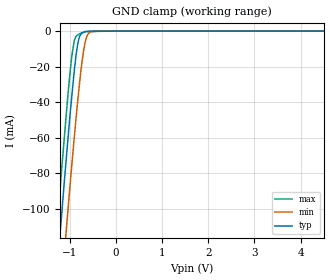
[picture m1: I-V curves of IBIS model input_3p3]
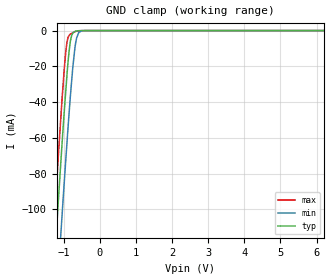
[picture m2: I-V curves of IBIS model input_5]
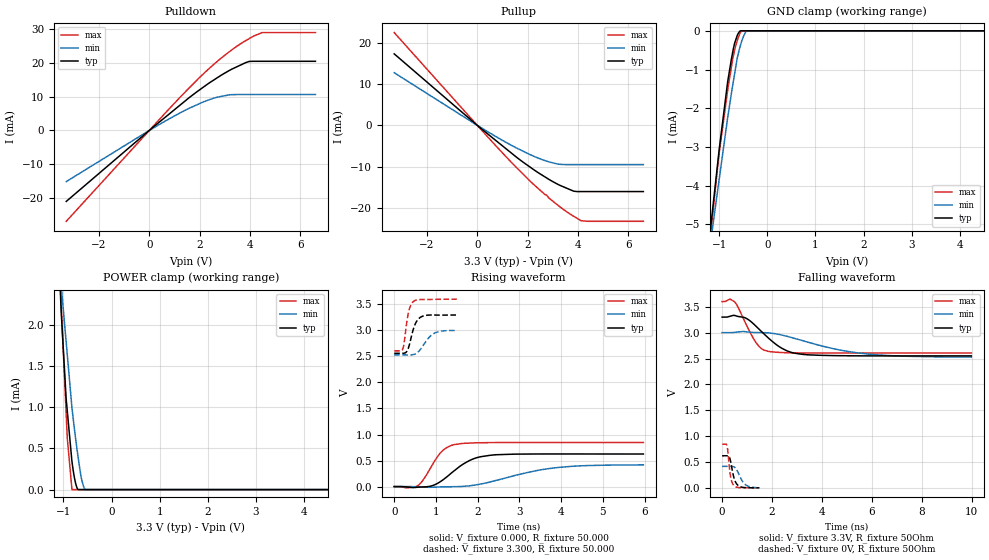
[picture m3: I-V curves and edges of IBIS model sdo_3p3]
|Texas Instruments Incorporated
| 2.7V-5.5V, 10 bit, 3MSPS, Serial ADC
| Marketing part#   Digital Voltage Range   Package-type   #pins
| ADS7884SDBVR   2.7V to 5.5V   SOT-23   6
| ADS7884SDBVT   2.7V to 5.5V   SOT-23   6
[IBIS Ver]   3.2
[File name]   ads7884.ibs
|SIMDE Ver   V3.0 - 201101 - RHL4 - Build 450
[File Rev]   1.0
[Date]   3/20/2011
[Source]
| Texas Instruments Incorporated.
| Analog-eLab Design Center, HPA
| 12500 TI Blvd
| Dallas, TX -75243
| e-mail: elab_ibis@list.ti.com
[Notes]   Revision History:
| Rev 1.0: 3/20/2011
| - Initial version of the model
| - Model generated from simulations in TISPICE
| - Model matched to SPICE simulation
| - C_comp although listed in numerical order of value are
|   obtained from varying PVT conditions. For PVT conditions for
|   each specific value refer the buffer description under
|   respective [Model]. IBIS model user is responsible for using
|   appropriate C_comp to simulate for Signal Integrity.
| - Model names with a trailing _3p3 contains the model for
|   3.3V [3.0V and 3.6V].Model names with a trailing _5 contains
|   the model for 5.0V [4.5V and 5.5V].
| - Rleative of ADS7883
[Disclaimer]
| This model is designed as an aid for customers of Texas Instruments.
| TI and its licensors and suppliers make no warranties, either expressed
| or implied, with respect to this  model, including the warranties of
| merchantability or fitness for a particular purpose. The model is
| provided solely on an "as is" basis. The entire risk as to its quality
| and performance is with the customer.
[Copyright]
 (C) Copyright 2011 Texas Instruments Incorporated.All rights reserved.
|   ADS7884
[Component]   ADS7884
[Manufacturer]   TI
[Package]   |6 SOT-23  -  DBV package
|   typ   min   max
R_pkg   0.00833   0.00820   0.00840
L_pkg   0.95512nH   0.93518nH   0.96766nH
C_pkg   0.21252pF   0.20183pF   0.24256pF
[Pin]  signal_name   model_name   R_pin   L_pin   C_pin
1   VDD   POWER   0.00811   0.93717nH  0.21052pF
2   GND   GND   0.00820   0.89025nH  0.21719pF
3   VIN   TERM   0.00840   0.96766nH  0.20183pF
4   SCLK   INPUT   0.00831   0.95468nH  0.20385pF
5   SDO   SDO   0.00820   0.93518nH  0.24256pF
6   _CS   INPUT   0.00840   0.96296nH  0.20183pF
|   Model Selectors
[Model Selector] INPUT
input_3p3   3.3V digital input
input_5   5.0V digital input
[Model Selector] SDO
sdo_3p3   3.3V digital 3-state output
sdo_5   5.0V digital 3-state output
[Model Selector] TERM
term_3-3V   3.3V nominal termination
term_5-0V   5.0V nominal termination
[Model]  term_3-3V
Model_type Terminator
C_comp   1.0e-20F  1.0e-20F  1.0e-20F
|   typ   min   max
[Voltage Range]   3.3V   3.0V   3.6V
[POWER Clamp Reference]   3.3V   3.0V   3.6V
[GND Clamp Reference]   0V   0V   0V
|Ambient Temperature   25   125   -40
|Junction Temperature
[Temperature Range]   30   130   -40
[Model]  term_5-0V
Model_type Terminator
C_comp   1.0e-20F  1.0e-20F  1.0e-20F
|   typ   min   max
[Voltage Range]   5.0V   4.5V   5.5V
[POWER Clamp Reference]   5.0V   4.5V   5.5V
[GND Clamp Reference]   0V   0V   0V
|Ambient Temperature   25   125   -40
|Junction Temperature
[Temperature Range]   30   130   -40
| Models and submodels in the file (6): input_3p3 (Input), input_5 (Input), sdo_3p3 (3-state), sdo_5 (3-state), term_3-3V (Terminator), term_5-0V (Terminator)
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|   input_3p3 Model
[Model]   input_3p3
Model_type   Input
Vinl = 0.4
Vinh = 1.5
|   typ   min   max
|   (nom PVT)   (Fast PVT)   (slow PVT)
|C_comp from frequency sweep method (F=48MHz)
|Average
C_comp   9.883e-13   8.635e-13   1.118e-12
|C_comp from LC tank measurement(L=1nH)
|Resonant Frequency(Hz)   5.810e+09   6.010e+09   5.610e+09
|C_comp   7.511e-13   7.020e-13   8.056e-13
| Where nom  PVT is Nominal Process,  3.3V,  30C
|   Fast PVT is Strong Process,   3.6V,  -40C
|   Slow PVT is Weak Process,   3V,  130C
[Voltage Range]   3.3   3   3.6
|Ambient Temperature   25   125   -40
|Junction Temperature
[Temperature Range]   30   130   -40
[Power Clamp Reference]   3.3   3   3.6
[GND Clamp Reference]   0   0   0
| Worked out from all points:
|   GND clamp passes 1 mA (typ) near -0.73 V on its own axis
[GND Clamp]
|   Voltage   I(typ)   I(min)   I(max)
-3.3V     -824.7mA   -854.6mA   -807mA
-1.294V   -141.5mA   -182mA     -117mA
-1.167V   -100.8mA   -140.8mA   -75.49mA
-1.115V   -84.28mA   -124.8mA   -59.63mA
-1.037V   -60.45mA   -100.3mA   -35.47mA
-954mV    -36.58mA   -75.2mA    -13.96mA
-896.4mV  -21.14mA   -58.46mA   -4.929mA
-802.8mV  -4.674mA   -33.3mA    -1.741mA
-741mV    -1.172mA   -18.82mA   -1.098mA
-666mV    -306.2uA   -6.367mA   -434.3uA
-540mV    -191.2uA   -375.4uA   -33.33uA
6.6V      0A         0A         0A
[POWER Clamp]
|   Voltage   I(typ)   I(min)   I(max)
-3.3V     0A         0A         0A
6.6V      0A         0A         0A
|   input_5 Model
[Model]   input_5
Model_type   Input
Vinl = 0.8
Vinh = 2.2
|   typ   min   max
|   (nom PVT)   (Fast PVT)   (slow PVT)
|C_comp from frequency sweep method (F=48MHz)
|Average
C_comp   9.397e-13   8.279e-13   1.058e-12
|C_comp from LC tank measurement(L=1nH)
|Resonant Frequency(Hz)   5.880e+09   6.070e+09   5.700e+09
|C_comp   7.334e-13   6.882e-13   7.804e-13
| Where nom  PVT is Nominal Process,  5V,  30C
|   Fast PVT is Strong Process,   5.5V,  -40C
|   Slow PVT is Weak Process,   4.5V,  130C
[Voltage Range]   5   4.5   5.5
|Ambient Temperature   25   125   -40
|Junction Temperature
[Temperature Range]   30   130   -40
[Power Clamp Reference]   5   4.5   5.5
[GND Clamp Reference]   0   0   0
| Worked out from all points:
|   GND clamp passes 1 mA (typ) near -0.74 V on its own axis
[GND Clamp]
|   Voltage   I(typ)   I(min)   I(max)
-5V       -1.412A    -1.436A    -1.399A
-1.368V   -166mA     -205.4mA   -141.5mA
-1.188V   -107.6mA   -147.5mA   -82.23mA
-1.127V   -88.16mA   -128.6mA   -62.97mA
-1.05V    -64.35mA   -104.5mA   -39.47mA
-979mV    -43.28mA   -82.7mA    -19.79mA
-913mV    -25.38mA   -63.22mA   -6.748mA
-815mV    -5.773mA   -36.27mA   -1.956mA
-670mV    -322.9uA   -6.853mA   -476uA
-580.5mV  -63.28uA   -988.6uA   -181.1uA
-373.5mV  -1.333uA   -5.052uA   -6.916uA
10V       0A         0A         0A
[POWER Clamp]
|   Voltage   I(typ)   I(min)   I(max)
-5V       0A         0A         0A
10V       0A         0A         0A
|   sdo_3p3 Model
[Model]   sdo_3p3
Model_type   3-state
Polarity   Non-Inverting
Vmeas = 1.65
Vref = 1.65
Cref = 10pF
Rref = 50
|   typ   min   max
|   (nom PVT)   (Fast PVT)   (slow PVT)
|C_comp from frequency sweep method(F=48MHz)
|C_comp   9.342e-13   8.281e-13   1.130e-12
|ON state : BUFFER OUTPUT TURNED HIGH
|C_comp   9.342e-13   8.281e-13   1.130e-12
|OFF state: BUFFER IN HIGH IMPEDANCE
|C_comp   1.178e-12   9.982e-13   1.365e-12
|C_comp from LC tank measurement(L=1nH)
|Resonant Frequency(Hz)   6.460e+09   6.710e+09   6.330e+09
C_comp   6.076e-13   5.632e-13   6.328e-13
|ON state : BUFFER OUTPUT TURNED HIGH
|Resonant Frequency(Hz)   6.460e+09   6.710e+09   6.330e+09
|C_comp   6.076e-13   5.632e-13   6.328e-13
|OFF state: BUFFER IN HIGH IMPEDANCE
|Resonant Frequency   6.110e+09   6.600e+09   5.830e+09
|C_comp   6.792e-13   5.821e-13   7.460e-13
| Where nom  PVT is Nominal Process,  3.3V,  30C
|   Fast PVT is Strong Process,   3.6V,  -40C
|   Slow PVT is Weak Process,   3V,  130C
[Voltage Range]   3.3   3   3.6
|Ambient Temperature   25   125   -40
|Junction Temperature
[Temperature Range]   30   130   -40
[Pullup Reference]   3.3   3   3.6
[Pulldown Reference]   0   0   0
[Power Clamp Reference]   3.3   3   3.6
[GND Clamp Reference]   0   0   0
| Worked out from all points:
|   slope of the pulldown table from 0 to 0.495 V, typ, clamps not added: 162 ohm
|   slope of the pullup table from 0 to 0.495 V, typ, clamps not added: 200 ohm
|   GND clamp passes 1 mA (typ) near -0.78 V on its own axis
|   POWER clamp passes 1 mA (typ) near -0.93 V on its own axis
|   falling waveform, V_fixture 3.3V, R_fixture 50Ohm: 20-80 % time 1.08ns typ, 2.46ns min, 635ps max; typ from 3.3 V to 2.55 V
|   rising waveform, V_fixture 0.000, R_fixture 50.000: 20-80 % time 644ps typ, 1.33ns min, 413ps max; typ from 0 V to 0.625 V
|   rising waveform, V_fixture 3.300, R_fixture 50.000: 20-80 % time 162ps typ, 272ps min, 114ps max; typ from 2.56 V to 3.29 V
|   falling waveform, V_fixture 0V, R_fixture 50Ohm: 20-80 % time 180ps typ, 287ps min, 123ps max; typ from 0.621 V to 0.002 V
[Pulldown]
|   Voltage   I(typ)   I(min)   I(max)
-3.3V     -21.06mA   -15.19mA   -26.96mA
0V        0A         0A         0A
1.29V     7.925mA    5.45mA     10.38mA
2.277V    13.53mA    8.822mA    17.68mA
2.7V      15.62mA    9.857mA    20.48mA
3.27V     18.14mA    10.6mA     23.86mA
3.97V     20.45mA    10.65mA    27.23mA
4.483V    20.49mA    10.65mA    29.02mA
6.6V      20.49mA    10.65mA    29.02mA
[GND Clamp]
|   Voltage   I(typ)   I(min)   I(max)
-3.3V     -31.86mA   -26.3mA    -39mA
-1.18V    -5.077mA   -5.443mA   -5.263mA
-1.01V    -3.162mA   -3.913mA   -3.234mA
-825mV    -1.313mA   -2.237mA   -1.529mA
-726mV    -584.3uA   -1.442mA   -763.6uA
-683.1mV  -331.7uA   -1.122mA   -511uA
-630mV    -133.7uA   -725.1uA   -269.5uA
-567.6mV  -2.719uA   -407.5uA   -62.56uA
-535.2mV  0A         -273.4uA   0A
-486mV    0A         -111.5uA   0A
-438mV    0A         -1.634uA   0A
6.6V      0A         0A         0A
[Pullup]
|   Voltage   I(typ)   I(min)   I(max)
-3.3V     17.35mA    12.77mA    22.52mA
0V        0A         0A         0A
1.149V    -5.708mA   -4.153mA   -7.649mA
1.574V    -7.808mA   -5.548mA   -10.34mA
2.277V    -10.9mA    -7.585mA   -14.55mA
2.7V      -12.56mA   -8.577mA   -16.85mA
2.755V    -12.76mA   -8.682mA   -16.91mA
2.842V    -13.1mA    -8.851mA   -17.62mA
3.205V    -14.33mA   -9.386mA   -19.41mA
3.831V    -15.98mA   -9.532mA   -22.07mA
4.134V    -16.08mA   -9.532mA   -23.17mA
6.6V      -16.08mA   -9.532mA   -23.29mA
[POWER Clamp]
|   Voltage   I(typ)   I(min)   I(max)
-3.3V     43.14mA    33.87mA    53.61mA
-1.143V   3.495mA    3.12mA     4.243mA
-1.049V   2.194mA    2.498mA    2.361mA
-1.036V   2.045mA    2.406mA    2.099mA
-943.8mV  1.104mA    1.795mA    926.4uA
-920.4mV  955.6uA    1.64mA     627.4uA
-823.2mV  344uA      996.3uA    0A
-759mV    107.9uA    676.4uA    0A
-706.2mV  6.277uA    441.7uA    0A
-630mV    0A         145.2uA    0A
-555mV    0A         31.3nA     0A
6.6V      0A         0A         0A
[Ramp]
R_load = 50
|   typ   min   max
dV/dt_r   0.37497/6.43447e-10   0.250507/1.33256e-09   0.5127/4.11078e-10
dV/dt_f   0.449324/1.08338e-09   0.283649/2.45466e-09   0.595524/6.34571e-10
[Falling Waveform]
V_fixture = 3.3V
V_fixture_min = 3V
V_fixture_max = 3.6V
R_fixture = 50Ohm
|   Time   V(typ)   V(min)   V(max)
0s        3.3V       3V         3.6V
310ps     3.315V     3V         3.647V
510ps     3.331V     3.005V     3.588V
960ps     3.278V     3.017V     3.162V
1.34ns    3.132V     3.002V     2.822V
1.86ns    2.894V     2.995V     2.637V
2.6ns     2.648V     2.929V     2.612V
3.29ns    2.577V     2.836V     2.606V
5.88ns    2.551V     2.584V     2.606V
9.99ns    2.551V     2.527V     2.607V
[Rising Waveform]
V_fixture = 0.000
V_fixture_min = 0.000
V_fixture_max = 0.000
R_fixture = 50.000
|  time   V(typ)   V(min)   V(max)
0s        -2.813uV   8.632uV    0V
310ps     -7.985mV   158.5uV    -24.09mV
570ps     -11.73mV   -4.704mV   21.65mV
720ps     -6.205mV   -10.13mV   158mV
1.09ns    85.97mV    -6.545mV   631.3mV
1.45ns    311.3mV    -1.882mV   808.3mV
1.87ns    524mV      21.68mV    838.1mV
2.41ns    610mV      111.9mV    845.3mV
3.9ns     626.5mV    364.6mV    846mV
5.97ns    625.4mV    417.1mV    845.4mV
[Rising Waveform]
V_fixture = 3.300
V_fixture_min = 3.000
V_fixture_max = 3.600
R_fixture = 50.000
|  time   V(typ)   V(min)   V(max)
0s        2.559V     2.529V     2.606V
205ps     2.56V      2.529V     2.644V
235ps     2.562V     2.529V     2.746V
307ps     2.599V     2.528V     3.187V
346ps     2.675V     2.528V     3.357V
403ps     2.854V     2.529V     3.493V
478ps     3.069V     2.54V      3.565V
643ps     3.259V     2.65V      3.594V
955ps     3.295V     2.942V     3.595V
1.498ns   3.295V     2.998V     3.6V
[Falling Waveform]
V_fixture = 0V
V_fixture_min = 0V
V_fixture_max = 0V
R_fixture = 50Ohm
|   Time   V(typ)   V(min)   V(max)
0s        621.2mV    416.6mV    845.4mV
193ps     621.8mV    416.4mV    820.7mV
229ps     621mV      416.4mV    712mV
277ps     605.9mV    416.6mV    463.9mV
337ps     521.5mV    417.1mV    225.9mV
394ps     377mV      416.2mV    112.3mV
469ps     205.9mV    407.5mV    47.51mV
637ps     49.52mV    300.6mV    9.065mV
937ps     5.18mV     63.17mV    2.442mV
1.498ns   1.922mV    3.016mV    1.249mV
